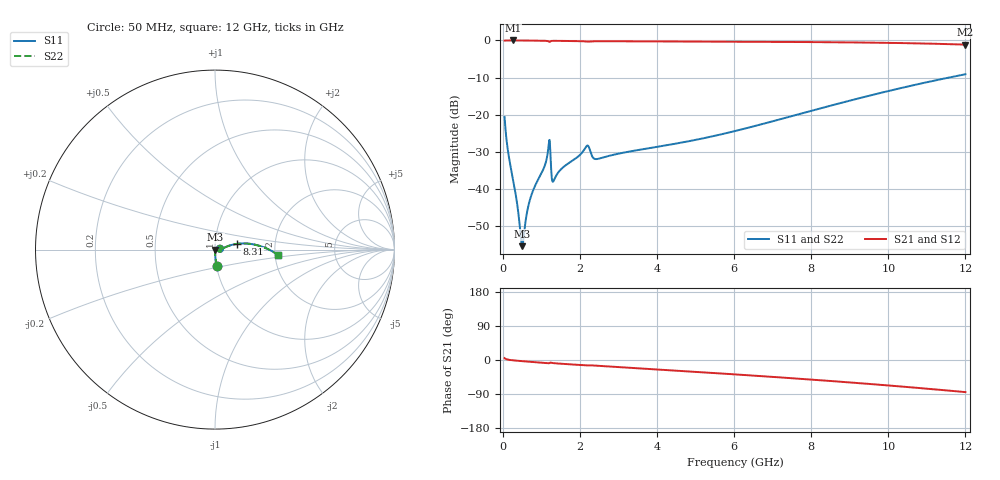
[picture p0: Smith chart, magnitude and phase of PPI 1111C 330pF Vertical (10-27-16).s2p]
# GHz S MA R 50
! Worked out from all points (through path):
!   1601 points, 50 MHz to 12 GHz, reference 50 ohm
!   highest |S21| = 0.00 dB at 266.6 MHz (marker M1); lowest = -1.1 dB at 12 GHz (marker M2)
!   group delay of S21, straight-line fit = 19.2 ps
!   lowest |S11| = -55.5 dB at 505.6 MHz (marker M3), VSWR 1.00, Z = 50.2 - j0.0464 ohm
!   |S11| at or under -10 dB: start of sweep to 11.58 GHz
!   |S22| runs from -55.5 to -9.1 dB; largest |S21 - S12| = 0
!   S11 on the Smith chart (normalised r, x): 50 MHz: 1.00, -0.19; 8.31 GHz: 1.27, +0.08; 12 GHz: 2.06, -0.13
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0.05  0.09247 -84.6  0.995 5.0  0.995 5.0  0.09247 -84.6
0.1545625  0.02818 -88.2  0.9991 0.7  0.9991 0.7  0.02818 -88.2
0.2665938  0.01346 -88.9  0.9994 -0.8  0.9994 -0.8  0.01346 -88.9
0.3636875  0.006864 -85.9  0.9992 -1.8  0.9992 -1.8  0.006864 -85.9
0.4607812  0.002509 -62.1  0.9987 -2.7  0.9987 -2.7  0.002509 -62.1
0.5055937  0.001678 -16.0  0.9983 -3.1  0.9983 -3.1  0.001678 -16.0
0.5429375  0.002203 23.1  0.998 -3.4  0.998 -3.4  0.002203 23.1
0.6400313  0.005077 49.8  0.997 -4.1  0.997 -4.1  0.005077 49.8
0.7221875  0.007548 53.3  0.9959 -4.8  0.9959 -4.8  0.007548 53.3
1.073219  0.01929 50.2  0.9895 -7.4  0.9895 -7.4  0.01929 50.2
1.177781  0.03324 40.8  0.978 -8.6  0.978 -8.6  0.03324 40.8
1.215125  0.04554 5.5  0.9556 -8.0  0.9556 -8.0  0.04554 5.5
1.327156  0.01296 17.0  0.9882 -8.4  0.9882 -8.4  0.01296 17.0
2.044156  0.03004 26.0  0.9765 -13.5  0.9765 -13.5  0.03004 26.0
2.201  0.03822 8.8  0.9646 -14.2  0.9646 -14.2  0.03822 8.8
2.447469  0.02513 5.6  0.9763 -15.3  0.9763 -15.3  0.02513 5.6
4.038312  0.03694 8.0  0.9687 -25.3  0.9687 -25.3  0.03694 8.0
6.025  0.05993 13.3  0.9611 -38.0  0.9611 -38.0  0.05993 13.3
8.019156  0.1129 15.3  0.9502 -51.8  0.9502 -51.8  0.1129 15.3
8.310438  0.124 14.8  0.9479 -53.9  0.9479 -53.9  0.124 14.8
10.01331  0.2084 8.4  0.9274 -67.3  0.9274 -67.3  0.2084 8.4
12  0.3497 -4.6  0.8783 -84.7  0.8783 -84.7  0.3497 -4.6
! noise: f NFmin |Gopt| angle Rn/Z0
0.05  0.0005737  0.911  0.3271  0.001419
1.372  0.0124  0.8889  8.316  0.02414
2.701  0.0248  0.8918  16.28  0.04893
4.031  0.03392  0.8849  24.06  0.06121
5.36  0.04143  0.8787  31.6  0.06841
6.682  0.04818  0.8747  38.81  0.07384
8.012  0.05473  0.873  45.73  0.07899
9.341  0.06134  0.8737  52.3  0.08451
10.67  0.06826  0.8763  58.51  0.09085
12  0.07569  0.8805  64.37  0.09843
